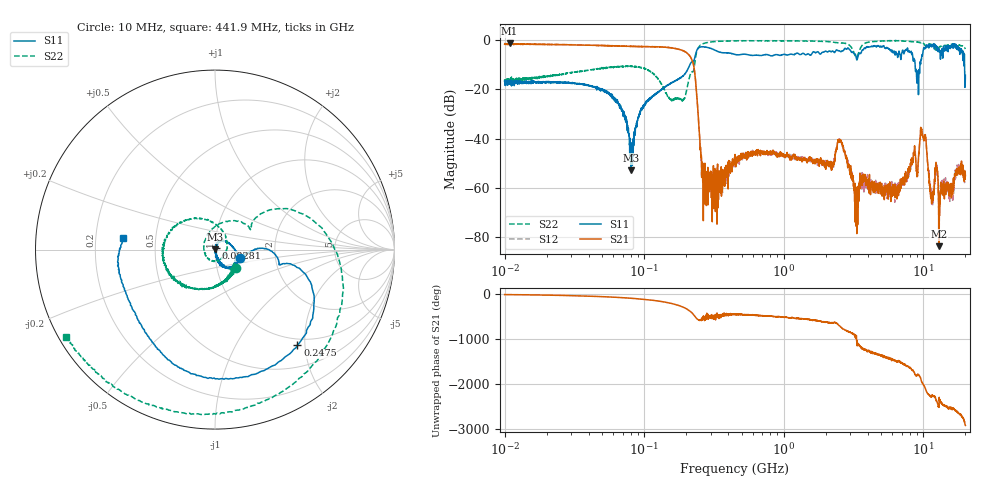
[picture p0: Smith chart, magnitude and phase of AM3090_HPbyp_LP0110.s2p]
# Hz S DB R 50
!freq MagS11 AngS11 MagS21 AngS21 MagS12 AngS12 MagS22 AngS22
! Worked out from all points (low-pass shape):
!   3201 points, 10 MHz to 20 GHz, reference 50 ohm
!   highest |S21| = -1.43 dB at 10.84 MHz (marker M1); lowest = -83.6 dB at 12.89 GHz (marker M2)
!   |S21| within 3 dB of the highest: start of sweep to 190.6 MHz; 190.7215 MHz to 191.4029 MHz (681.4 kHz wide, 0.357 % of centre)
!   lowest |S11| = -52.9 dB at 80.68 MHz (marker M3), VSWR 1.00, Z = 50.2 + j0.151 ohm
!   |S11| at or under -10 dB: start of sweep to 212.5 MHz; 8.728 GHz to 9.453 GHz (724.4 MHz wide, 7.97 % of centre); 19.73 GHz to end of sweep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
!   |S22| runs from -24.8 to -0.2 dB; largest |S21 - S12| = 0.034
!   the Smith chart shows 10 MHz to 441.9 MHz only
!   S11 on the Smith chart (normalised r, x): 10 MHz: 1.31, -0.13; 82.81 MHz: 1.01, +0.02; 247.5 MHz: 0.88, -1.85; 441.9 MHz: 0.32, +0.05
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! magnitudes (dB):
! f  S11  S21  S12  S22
! 10 MHz  -16.7  -1.7  -1.6  -16.1
! 10.84 MHz  -17.1  -1.4  -1.6  -16.5
! 35.55 MHz  -17.9  -2.1  -2.0  -12.7
! 63.77 MHz  -25.0  -2.4  -2.4  -10.9
! 80.68 MHz  -52.9  -2.6  -2.5  -10.7
! 82.81 MHz  -40.2  -2.6  -2.6  -10.7
! 126.1 MHz  -21.3  -2.8  -2.8  -15.8
! 187 MHz  -14.9  -4.2  -4.2  -24.2
! 216.7 MHz  -9.2  -7.3  -7.3  -13.3
! 247.5 MHz  -3.1  -36.9  -36.5  -2.6
! 271.6 MHz  -2.8  -53.3  -58.0  -1.3
! 441.9 MHz  -5.8  -48.5  -50.8  -0.3
! 447.2 MHz  -5.9  -46.5  -48.1  -0.3
! 1.59 GHz  -5.5  -49.4  -48.2  -0.4
! 2.521 GHz  -4.5  -40.5  -40.8  -1.2
! 3.328 GHz  -8.0  -66.0  -70.0  -7.1
! 5.639 GHz  -3.7  -61.5  -63.4  -0.3
! 9.09 GHz  -14.4  -53.6  -52.5  -0.9
! 9.901 GHz  -5.2  -39.0  -38.9  -1.3
! 11.44 GHz  -2.8  -64.8  -66.3  -1.9
! 12.89 GHz  -3.8  -83.6  -65.6  -3.1
! 20 GHz  -14.4  -55.0  -53.5  -3.7
